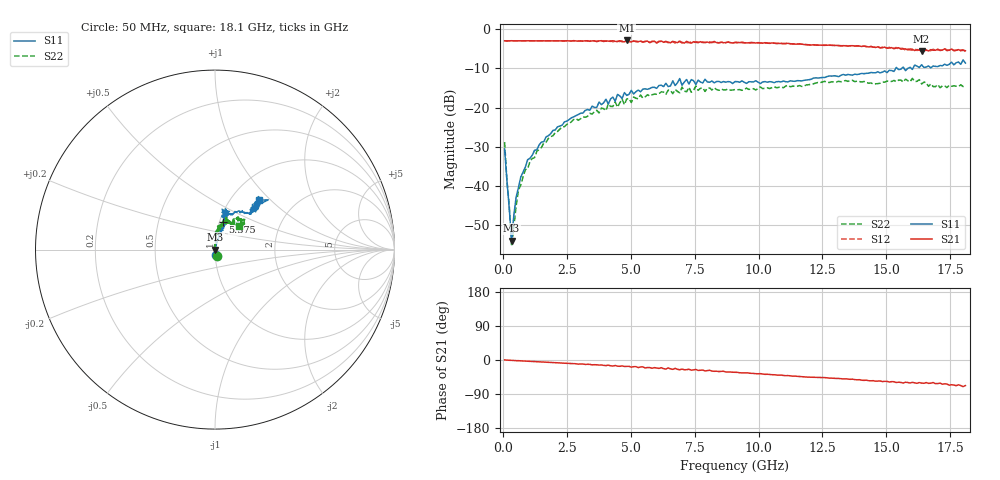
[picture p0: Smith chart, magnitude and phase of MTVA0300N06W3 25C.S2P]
! Network Analyzer HP8720D.06.14 Serial No. US36140669
!  7 Jul 2005  10:02:57
! Frequency  S11  S21  S12  S22
# HZ  S  DB R 50
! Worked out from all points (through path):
!   201 points, 50 MHz to 18.1 GHz, reference 50 ohm
!   highest |S21| = -2.87 dB at 4.833 GHz (marker M1); lowest = -5.6 dB at 16.39 GHz (marker M2)
!   group delay of S21, straight-line fit = 10.5 ps
!   lowest |S11| = -53.9 dB at 320.8 MHz (marker M3), VSWR 1.00, Z = 50.2 + j0.0288 ohm
!   |S11| at or under -10 dB: start of sweep to 15.37 GHz; 15.43 GHz to 15.61 GHz (171.9 MHz wide, 1.11 % of centre); 15.7 GHz to 15.84 GHz (145.4 MHz wide, 0.922 % of centre)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
!   |S22| runs from -55.3 to -12.5 dB; largest |S21 - S12| = 0.037
!   S11 on the Smith chart (normalised r, x): 50 MHz: 1.01, -0.06; 5.375 GHz: 1.04, +0.33; 18.1 GHz: 1.34, +0.86
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5e7  -30.53 -78.5  -2.96 0.2  -2.94 0.1  -28.78 -69.1
1.4025e8  -38.59 -73.2  -2.99 -0.4  -2.98 -0.4  -38.54 -90.5
2.305e8  -45.47 -57.1  -2.95 -0.7  -2.95 -0.7  -44.87 -102.3
3.2075e8  -53.90 8.2  -2.94 -0.9  -2.96 -0.9  -55.34 -147.1
5.0125e8  -42.84 74.0  -2.96 -1.8  -2.96 -1.7  -45.12 107.6
5.915e8  -40.40 77.7  -2.96 -1.8  -2.98 -1.9  -41.02 106.9
9.525e8  -33.28 77.4  -2.96 -3.2  -2.95 -3.2  -35.59 98.5
1.76475e9  -27.18 77.6  -2.95 -6.1  -2.96 -6.2  -27.87 88.1
3.1185e9  -21.38 73.9  -3.03 -10.5  -3.05 -10.9  -22.35 87.6
4.83325e9  -16.89 77.0  -2.87 -16.8  -3.10 -17.8  -17.80 74.3
5.37475e9  -15.94 73.9  -3.04 -18.2  -3.04 -19.2  -16.78 76.7
6.09675e9  -14.35 71.8  -3.15 -22.2  -3.07 -21.9  -16.44 73.2
6.7285e9  -14.37 78.5  -3.26 -22.1  -3.51 -23.2  -15.39 67.0
6.909e9  -12.59 75.5  -3.04 -25.8  -3.18 -24.0  -16.23 66.9
6.99925e9  -14.29 75.3  -3.37 -24.0  -3.49 -26.1  -14.77 67.5
7.17975e9  -12.83 80.0  -3.09 -25.5  -3.40 -24.3  -15.96 62.9
7.54075e9  -14.10 72.0  -3.34 -24.9  -3.17 -27.7  -14.50 70.8
9.075e9  -13.36 75.2  -3.38 -32.3  -3.35 -32.4  -15.40 60.9
1.21435e10  -12.48 62.0  -3.99 -45.3  -3.95 -45.4  -13.93 58.0
1.512175e10  -10.47 44.8  -4.80 -58.1  -4.61 -57.4  -13.33 53.0
1.638525e10  -9.07 45.0  -5.61 -61.0  -5.29 -59.9  -13.97 44.1
1.81e10  -8.63 48.1  -5.48 -67.6  -5.73 -68.7  -14.52 43.5
